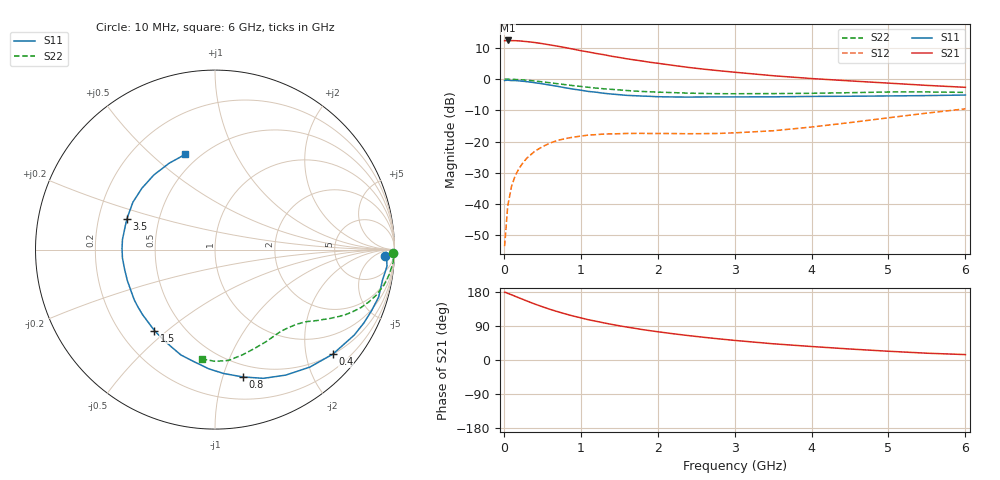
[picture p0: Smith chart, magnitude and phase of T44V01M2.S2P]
! Infineon Technologies  Discrete & RF Semiconductors
! BFR182T
! Si NPN RF Bipolar Junction Transistor in SC75
! VCE = 4 V  IC = 1.2 mA
! Common Emitter S-Parameters:  October  1999
# GHz  S  MA  R  50
!  f  S11  S21  S12  S22
! GHz  MAG  ANG  MAG  ANG  MAG  ANG  MAG  ANG
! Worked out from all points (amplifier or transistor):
!   36 points, 10 MHz to 6 GHz, reference 50 ohm
!   highest |S21| = 12.4 dB at 50 MHz (marker M1)
!   |S21| within 3 dB of that: start of sweep to 944.9 MHz
!   unconditionally stable (mu >= 1): 2.311 GHz to 4.505 GHz
!   at 250 MHz: K = 0.11, MSG = 19.5 dB, |S12| = -26.8 dB
!   at 1.4 GHz: K = 0.62, MSG = 12.5 dB, |S12| = -17.6 dB
!   at 6 GHz: K = 0.83, MSG = 3.5 dB, |S12| = -9.5 dB
!   S11 on the Smith chart (normalised r, x): 10 MHz: 25, -17; 400 MHz: 0.50, -2.55; 800 MHz: 0.39, -1.17; 1.5 GHz: 0.34, -0.45; 3.5 GHz: 0.32, +0.15; 6 GHz: 0.42, +0.65
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0.01  0.9476 -2.1  4.137 178.6  0.0021 79.6  0.9905 -1.2
0.02  0.9548 -0.9  4.132 178.7  0.003 89.7  0.9999 -0.9
0.05  0.9628 -5.5  4.169 175.9  0.0092 91.7  0.9957 -2.1
0.1  0.9486 -10.3  4.138 172.2  0.0191 83.4  0.9948 -4.2
0.15  0.9493 -16.2  4.133 167.9  0.0287 80.6  0.9865 -6.3
0.25  0.9247 -26.2  4.048 159.8  0.0458 74.2  0.9709 -10.3
0.4  0.8776 -41.6  3.867 147.8  0.0695 66.5  0.9335 -15.8
0.5  0.8412 -51.1  3.707 140.7  0.0824 61.4  0.9051 -18.8
0.6  0.8027 -60.6  3.539 133.7  0.0944 56.8  0.8746 -21.7
0.7  0.7662 -69.4  3.369 127.5  0.1044 52.5  0.8439 -24.1
0.8  0.7265 -77.6  3.204 121.6  0.1113 49.0  0.8152 -26.3
0.9  0.692 -86.0  3.029 116.1  0.1174 45.8  0.7868 -28.2
1.1  0.6347 -100.8  2.725 106.2  0.1268 40.9  0.7402 -31.4
1.3  0.5933 -114.4  2.465 98.0  0.1318 37.3  0.7004 -34.2
1.5  0.5635 -126.8  2.225 90.4  0.1334 34.9  0.6716 -36.4
1.8  0.5349 -143.6  1.95 80.3  0.1351 32.9  0.6342 -39.9
2.2  0.5179 -160.7  1.662 69.3  0.1342 33.5  0.6076 -44.2
2.8  0.5181 179.4  1.363 55.7  0.1348 39.0  0.5843 -52.0
3.5  0.5201 161.0  1.134 42.8  0.1487 48.8  0.5866 -61.1
4.5  0.5318 140.0  0.937 29.0  0.201 58.5  0.6064 -75.5
5.5  0.5448 118.0  0.794 17.9  0.2855 59.4  0.6226 -89.9
6  0.5559 107.4  0.739 14.3  0.3339 56.8  0.6133 -96.7
